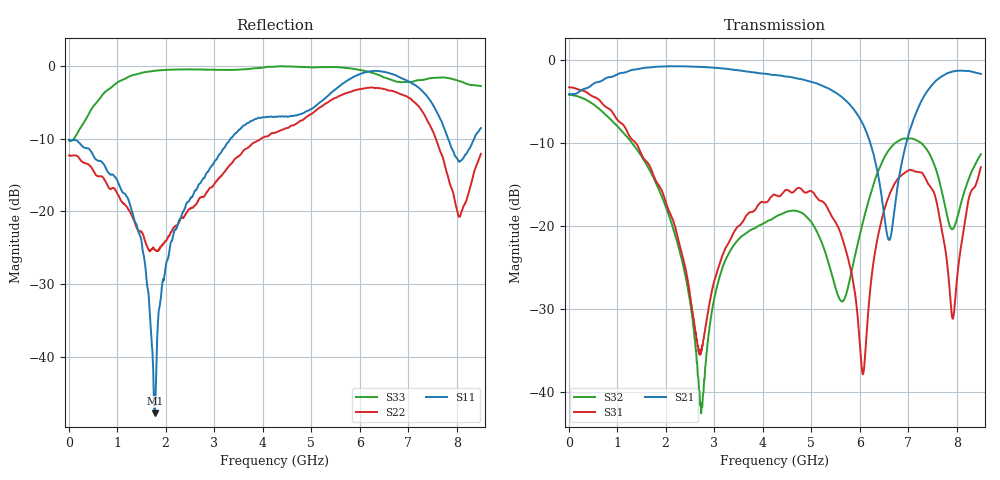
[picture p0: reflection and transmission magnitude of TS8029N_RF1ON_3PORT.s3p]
!Created with skrf (http://scikit-rf.org).
# GHz S RI R 50.0
!freq ReS11 ImS11 ReS12 ImS12 ReS13 ImS13
! ReS21 ImS21 ReS22 ImS22 ReS23 ImS23
! ReS31 ImS31 ReS32 ImS32 ReS33 ImS33
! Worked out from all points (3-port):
!   1601 points, 10 MHz to 8.5 GHz, reference 50 ohm
!   strongest paths, dB at 10 MHz, 2.132 GHz, 4.255 GHz, 6.378 GHz, 8.5 GHz:
!     S21: -4.1, -0.7, -1.8, -13.7, -1.7
!     S31: -3.3, -19.0, -16.3, -21.2, -12.9
!     S32: -4.2, -19.9, -18.9, -13.4, -11.3
!   lowest |S11| = -47.8 dB at 1.782 GHz (marker M1), VSWR 1.01, Z = 50.3 - j0.277 ohm
!   |S11| at or under -10 dB: start of sweep to 3.34 GHz; 7.82 GHz to 8.364 GHz (543.7 MHz wide, 6.72 % of centre)
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0.01  -0.3104 0.00542  0.6228 0.00159  0.6859 -0.00977
      0.6226 0.00151  -0.2424 0.00423  0.6185 -0.01
      0.6857 -0.00987  0.6188 -0.00988  -0.3057 0.0165
1.246356  -0.022 0.1148  0.8335 -0.2173  0.0312 -0.3503
          0.8329 -0.2172  0.0374 0.0942  -0.00828 -0.3324
          0.0314 -0.3498  -0.0086 -0.3325  0.834 0.1285
1.782288  0.00301 -0.00275  0.7924 -0.4495  -0.0597 -0.1815
          0.7922 -0.4495  0.0453 -0.03  -0.1086 -0.1511
          -0.06 -0.1814  -0.1088 -0.151  0.8355 -0.3933
2.737413  -0.0861 -0.135  0.525 -0.7424  0.0109 -0.0138
          0.5248 -0.743  -0.1105 -0.0588  -0.00241 0.00763
          0.0109 -0.0139  -0.00239 0.00759  0.2722 -0.9029
4.255  -0.414 -0.1675  -0.0756 -0.8103  0.1122 -0.1058
       -0.076 -0.8094  -0.3317 0.0983  0.0836 -0.0756
       0.1117 -0.106  0.0838 -0.0756  -0.7501 -0.6395
5.533806  -0.6665 0.2214  -0.4373 -0.4514  -0.0227 -0.099
          -0.4381 -0.4514  -0.1364 0.5924  0.0159 -0.0362
          -0.0227 -0.099  0.0159 -0.0362  -0.8619 0.4656
6.069737  -0.6803 0.5775  -0.3693 -0.1779  -0.00949 0.00845
          -0.3694 -0.178  0.0884 0.6911  0.1055 0.0121
          -0.0095 0.00848  0.1055 0.0121  -0.6464 0.6664
6.552606  -0.3812 0.8171  -0.0659 -0.0661  0.1348 0.0299
          -0.0658 -0.0658  0.4847 0.4847  0.2496 -0.1093
          0.1347 0.0299  0.2501 -0.1095  -0.1092 0.8152
7.741206  0.2372 0.2876  -0.2295 -0.7801  -0.0552 -0.0575
          -0.2306 -0.7806  0.0434 -0.214  -0.0705 -0.1214
          -0.0551 -0.0576  -0.0702 -0.1216  0.8287 0.0261
8.5  -0.103 0.3586  -0.6696 -0.4816  0.2252 -0.0193
     -0.6701 -0.4813  -0.1731 0.1777  0.0991 -0.2517
     0.2253 -0.0197  0.0988 -0.2523  -0.1778 -0.7049
